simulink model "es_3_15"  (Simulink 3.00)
settings: Solver=ode1  SolverMode=SingleTasking  StartTime=0.0  StopTime=5  FixedStep=0.001  MaxStep=0.001  RelTol=1e-6  AbsTol=1e-6
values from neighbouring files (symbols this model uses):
  a = [0.5; 0.5; 0.5]    [inizia.M]
  q0 = pi*[1;-0.5;-0.5]    [inizia.M]
  Tc = 0.001    [inizia.M]
  Ts = @2;', 		'Mask Help','Implements a zeroth order discrete\nintegration using a gain, a sum, and\na unit delay. Inputs may be scalar\nor vector.\n')    [es_3_15.m]    (also in es_3_14.m; inizia.M = 0.002)

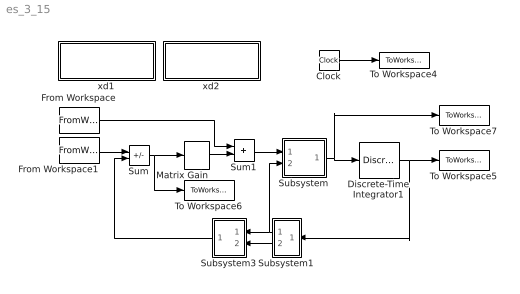
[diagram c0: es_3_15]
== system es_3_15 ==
  Clock : Clock
  Discrete-Time Integrator1 : DiscreteIntegrator  IntegratorMethod=ForwardEuler  ExternalReset=none  InitialConditionSource=internal  InitialCondition=q0  LimitOutput=off  UpperSaturationLimit=inf  LowerSaturationLimit=-inf  ShowSaturationPort=off  ShowStatePort=off  SampleTime=Tc
  From Workspace : FromWorkspace  VariableName=[T,dxd]  SampleTime=Tc  HoldFinalValue=off
  From Workspace1 : FromWorkspace  VariableName=[T,xd]  SampleTime=Tc  HoldFinalValue=off
  Matrix Gain : StateSpace  A=[]  B=[]  C=[]  D=K  X0=0  mask(Matrix Gain){}
      mask help: Matrix Gain.
      mask init:
      | K = @1;
  Subsystem : Subsystem
  Subsystem1 : Subsystem  Orientation=left
  Subsystem3 : Subsystem  Orientation=left
  Sum : Sum  Inputs=+-  SaturateOnIntegerOverflow=on
  Sum1 : Sum  Inputs=++  SaturateOnIntegerOverflow=on
  To Workspace4 : ToWorkspace  VariableName=time  SampleTime=Ts  SaveFormat=Matrix
  To Workspace5 : ToWorkspace  VariableName=qout  SampleTime=Ts  SaveFormat=Matrix
  To Workspace6 : ToWorkspace  VariableName=err  SampleTime=Ts  SaveFormat=Matrix
  To Workspace7 : ToWorkspace  VariableName=dqout  SampleTime=Ts  SaveFormat=Matrix
  xd1 : Subsystem
  xd2 : Subsystem
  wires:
  From Workspace1/1 -> Sum/1
  Matrix Gain/1 -> Sum1/2
  Sum1/1 -> Subsystem/1(in_1)
  From Workspace/1 -> Sum1/1
  Subsystem/1(out_1) -> Discrete-Time Integrator1/1, To Workspace7/1
  Sum/1 -> Matrix Gain/1, To Workspace6/1
  Discrete-Time Integrator1/1 -> To Workspace5/1, Subsystem1/1(in_1)
  Subsystem3/1(out_1) -> Sum/2
  Subsystem1/2(out_4) -> Subsystem3/2(iin_5)
  Subsystem1/1(out_5) -> Subsystem/2(in_2), Subsystem3/1(iin_4)
  Clock/1 -> To Workspace4/1

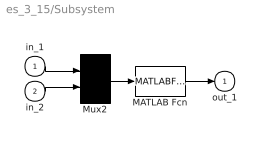
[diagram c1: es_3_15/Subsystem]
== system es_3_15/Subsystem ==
  in_1 : Inport  Port=1  PortWidth=-1  SampleTime=-1  DataType=auto
  in_2 : Inport  Port=2  PortWidth=-1  SampleTime=-1  DataType=auto
  MATLAB Fcn : MATLABFcn  MATLABFcn=invJa  OutputWidth=3  OutputSignalType=auto
  Mux2 : Mux  Inputs=[3,6]
  out_1 : Outport  Port=1  InitialOutput=0
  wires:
  Mux2/1 -> MATLAB Fcn/1
  in_1/1 -> Mux2/1
  MATLAB Fcn/1 -> out_1/1
  in_2/1 -> Mux2/2

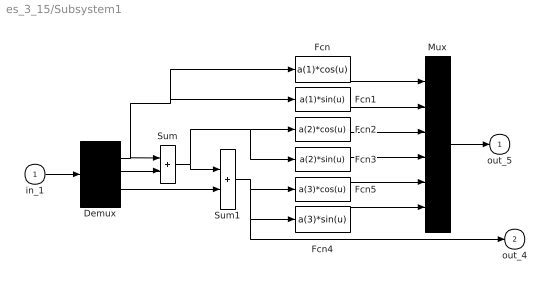
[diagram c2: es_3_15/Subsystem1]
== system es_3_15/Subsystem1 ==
  in_1 : Inport  Port=1  PortWidth=-1  SampleTime=-1  DataType=auto
  Demux : Demux  Outputs=3
  Fcn : Fcn  Expr=a(1)*cos(u)
  Fcn1 : Fcn  Expr=a(1)*sin(u)
  Fcn2 : Fcn  Expr=a(2)*cos(u)
  Fcn3 : Fcn  Expr=a(2)*sin(u)
  Fcn4 : Fcn  Expr=a(3)*sin(u)
  Fcn5 : Fcn  Expr=a(3)*cos(u)
  Mux : Mux  Inputs=6
  Sum : Sum  Inputs=++  SaturateOnIntegerOverflow=on
  Sum1 : Sum  Inputs=++  SaturateOnIntegerOverflow=on
  out_5 : Outport  Port=1  InitialOutput=0
  out_4 : Outport  Port=2  InitialOutput=0
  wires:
  in_1/1 -> Demux/1
  Demux/2 -> Sum/2
  Demux/3 -> Sum1/2
  Demux/1 -> Sum/1, Fcn/1, Fcn1/1
  Fcn/1 -> Mux/1
  Fcn1/1 -> Mux/2
  Fcn2/1 -> Mux/3
  Fcn3/1 -> Mux/4
  Fcn5/1 -> Mux/5
  Fcn4/1 -> Mux/6
  Sum1/1 -> Fcn5/1, Fcn4/1, out_4/1
  Mux/1 -> out_5/1
  Sum/1 -> Sum1/1, Fcn2/1, Fcn3/1

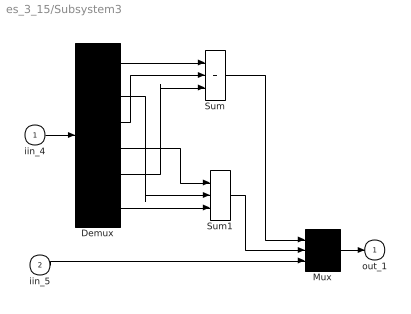
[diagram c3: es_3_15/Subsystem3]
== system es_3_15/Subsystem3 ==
  iin_4 : Inport  Port=1  PortWidth=-1  SampleTime=-1  DataType=auto
  iin_5 : Inport  Port=2  PortWidth=-1  SampleTime=-1  DataType=auto
  Demux : Demux  Outputs=6
  Mux : Mux  Inputs=3
  Sum : Sum  Inputs=+++  SaturateOnIntegerOverflow=on
  Sum1 : Sum  Inputs=+++  SaturateOnIntegerOverflow=on
  out_1 : Outport  Port=1  InitialOutput=0
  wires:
  iin_4/1 -> Demux/1
  Demux/1 -> Sum/1
  Demux/3 -> Sum/2
  Demux/5 -> Sum/3
  Demux/6 -> Sum1/3
  Demux/2 -> Sum1/2
  Demux/4 -> Sum1/1
  Sum1/1 -> Mux/2
  iin_5/1 -> Mux/3
  Sum/1 -> Mux/1
  Mux/1 -> out_1/1

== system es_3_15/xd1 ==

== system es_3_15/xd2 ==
